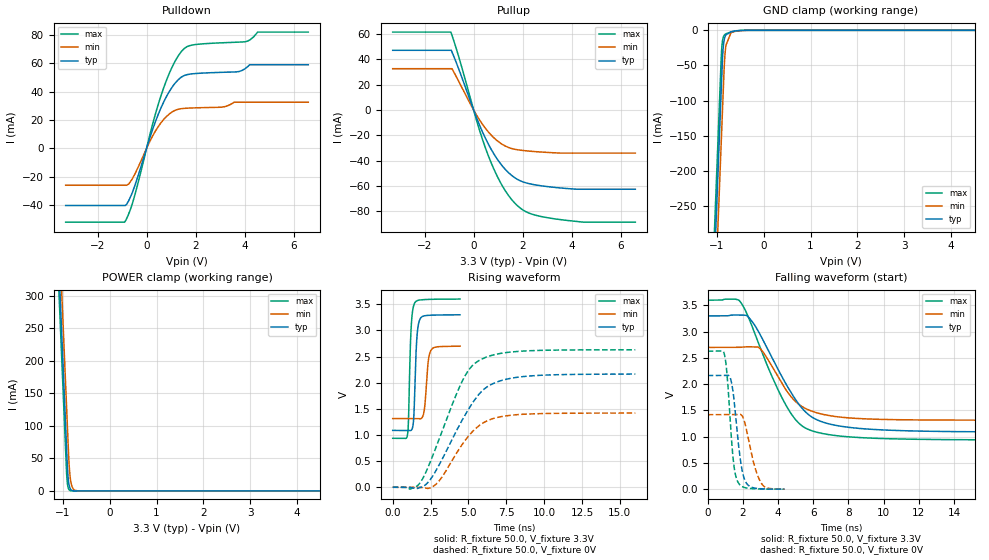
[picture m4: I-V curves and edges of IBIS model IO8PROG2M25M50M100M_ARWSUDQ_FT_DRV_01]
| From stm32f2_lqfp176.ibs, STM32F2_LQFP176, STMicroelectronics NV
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| *** New cell (Generated with 5.14beta1 (Sep 20 2010 13:23:23))
[Model]   IO8PROG2M25M50M100M_ARWSUDQ_FT_DRV_01
Model_type 3-state
Polarity   Non-Inverting
Enable   Active-Low
| CAP_THRESHOLD on pad IOV33 is "CMOS" :
| Rising=10.0% of vddio   Falling=90.0% of vddio
| C_comp min and max val. don't necessarily correlate with the min and max pvt
| but are the smallest and greatest pad capacitance found.
| var   typ   min   max
C_comp   2.32810pF  2.21815pF  2.46460pF
Vmeas = 1.65V   | Reference voltage for timing measurements
Cref  = 50.0pF   | Timing specification test load capacitance value
Rref  = 10.0MOhm   | Timing specification test load resistance value
Vref  = 1.65V   | Timing specification test load voltage
[Model Spec]
| variable   typ   min   max
[Temperature Range] 25.0 125.0 -40.0
| variable   typ   min   max
[Voltage Range] 3.3V 2.7V 3.6V
| variable   typ   min   max
[POWER Clamp Reference] 3.3V 2.7V 3.6V
| variable   typ   min   max
[GND Clamp Reference] 0V 0V 0V
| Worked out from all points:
|   slope of the pulldown table from 0 to 0.495 V, typ, clamps not added: 20 ohm
|   slope of the pullup table from 0 to 0.495 V, typ, clamps not added: 21.7 ohm
|   GND clamp passes 1 mA (typ) near -0.61 V on its own axis
|   POWER clamp passes 1 mA (typ) near -0.81 V on its own axis
|   rising waveform, R_fixture 50.0, V_fixture 3.3V: 20-80 % time 174ps typ, 219ps min, 160ps max; typ from 1.09 V to 3.3 V
|   falling waveform, R_fixture 50.0, V_fixture 3.3V: 20-80 % time 2.28ns typ, 1.77ns min, 2.12ns max; typ from 3.3 V to 1.09 V
|   rising waveform, R_fixture 50.0, V_fixture 0V: 20-80 % time 2.49ns typ, 2.07ns min, 2.18ns max; typ from 0 V to 2.17 V
|   falling waveform, R_fixture 50.0, V_fixture 0V: 20-80 % time 429ps typ, 610ps min, 343ps max; typ from 2.17 V to 0.001 V
[POWER Clamp]
-3.3V     4.11A      4.173A     4.072A
-1.09V    352.5mA    415.9mA    314.5mA
-1.05V    284.5mA    347.9mA    246.5mA
-1.01V    216.5mA    279.9mA    178.5mA
-920mV    63.51mA    126.9mA    25.85mA
-900mV    31.51mA    92.9mA     9.552mA
-890mV    21.35mA    75.9mA     5.807mA
-870mV    9.804mA    44.01mA    2.146mA
-840mV    3.05mA     18.36mA    482.1uA
-780mV    295.2uA    3.194mA    24.34uA
-660mV    2.764uA    96.52uA    62.42nA
6.6V      0A         0A         0A
[GND Clamp]
-3.3V     -4.149A    -4.224A    -4.103A
-1.06V    -341mA     -415.8mA   -295.1mA
-940mV    -137mA     -211.8mA   -91.11mA
-910mV    -86.01mA   -160.8mA   -40.11mA
-900mV    -69.01mA   -143.8mA   -27.13mA
-880mV    -37.2mA    -109.8mA   -14.07mA
-860mV    -20.02mA   -75.82mA   -8.837mA
-840mV    -11.77mA   -45.3mA    -6.542mA
-810mV    -6.468mA   -21.54mA   -4.94mA
-700mV    -2.247mA   -3.206mA   -2.168mA
-470mV    -130uA     -313.8uA   -60.76uA
6.6V      10.47nA    1.304uA    84.25pA
| variable   typ   min   max
[Pullup Reference] 3.3V 2.7V 3.6V
| variable   typ   min   max
[Pulldown Reference] 0V 0V 0V
[Pullup]
-3.3V     46.97mA    32.48mA    61.32mA
-930mV    46.97mA    32.48mA    61.32mA
-880mV    45.6mA     32.48mA    58.74mA
-590mV    31.42mA    21.88mA    40.86mA
240mV     -11.89mA   -7.822mA   -15.87mA
590mV     -26.5mA    -17.07mA   -35.52mA
1.18V     -44.36mA   -27.27mA   -60.11mA
1.54V     -51.43mA   -30.39mA   -70.35mA
1.89V     -55.75mA   -31.69mA   -77.18mA
2.48V     -58.98mA   -32.83mA   -82.75mA
3.6V      -61.62mA   -34.07mA   -86.61mA
6.6V      -62.54mA   -34.07mA   -88.51mA
[Pulldown]
-3.3V     -40.26mA   -25.94mA   -51.99mA
-870mV    -40.25mA   -25.94mA   -51.33mA
-720mV    -36.35mA   -24.93mA   -45.5mA
-470mV    -25.89mA   -17.87mA   -32.39mA
240mV     12.97mA    8.52mA     16.62mA
590mV     28.62mA    18.11mA    37.2mA
1.07V     43.85mA    26mA       58.31mA
1.54V     51.42mA    28.24mA    70.48mA
2.01V     52.82mA    28.63mA    73.27mA
4.01V     56.05mA    32.64mA    75.18mA
4.53V     59mA       32.64mA    82.02mA
6.6V      59mA       32.64mA    82.02mA
[Ramp]
dV/dt_r 1.29886V/2.48885ns 851.30659mV/2.0742ns 1.57728V/2.18503ns
dV/dt_f 1.32782V/2.27584ns 831.60247mV/1.77444ns 1.59819V/2.11818ns
R_load = 50.0
| Removed startup time: 0s 0s 0s  .
| Removed end time: 4.441ns.
[Rising Waveform]
R_fixture   = 50.0
V_fixture   = 3.3V
V_fixture_min = 2.7V
V_fixture_max = 3.6V
0s        1.087V     1.314V     936.3mV
980ps     1.087V     1.314V     1.006V
1.042ns   1.086V     1.314V     1.284V
1.208ns   1.086V     1.314V     3V
1.429ns   1.589V     1.314V     3.511V
1.587ns   2.822V     1.313V     3.564V
1.809ns   3.219V     1.309V     3.581V
2.085ns   3.278V     1.472V     3.588V
2.521ns   3.29V      2.617V     3.594V
4.443ns   3.298V     2.698V     3.598V
| Removed startup time: 0s 0s 0s  .
| Removed end time: 20.415ns.
[Falling Waveform]
R_fixture   = 50.0
V_fixture   = 3.3V
V_fixture_min = 2.7V
V_fixture_max = 3.6V
0s        3.3V       2.7V       3.6V
1.83ns    3.315V     2.701V     3.579V
2.28ns    3.29V      2.711V     3.304V
2.955ns   2.962V     2.685V     2.725V
4.335ns   2.073V     1.953V     1.67V
5.02ns    1.694V     1.661V     1.315V
5.735ns   1.419V     1.51V      1.135V
6.95ns    1.239V     1.399V     1.036V
9.1ns     1.144V     1.337V     975.1mV
20.43ns   1.087V     1.314V     936.6mV
| Removed startup time: 0s 0s 0s  .
| Removed end time: 16.01ns.
[Rising Waveform]
R_fixture   = 50.0
V_fixture   = 0V
V_fixture_min = 0V
V_fixture_max = 0V
0s        8.041nV    322.2nV    5.734nV
1.14ns    -513.1uV   -6.917uV   -36.27mV
1.85ns    -3.412mV   -2.228mV   102.7mV
2.345ns   97.24mV    -22.08mV   389.7mV
2.97ns    376.1mV    89.52mV    846.8mV
4.63ns    1.306V     835.3mV    2.051V
5.79ns    1.809V     1.195V     2.439V
6.75ns    1.999V     1.324V     2.538V
8.385ns   2.109V     1.391V     2.6V
16.02ns   2.165V     1.419V     2.629V
| Removed startup time: 0s 0s 0s  .
| Removed end time: 4.359ns.
[Falling Waveform]
R_fixture   = 50.0
V_fixture   = 0V
V_fixture_min = 0V
V_fixture_max = 0V
0s        2.165V     1.419V     2.629V
965ps     2.166V     1.419V     2.552V
1.146ns   2.171V     1.419V     2.02V
1.364ns   2.019V     1.418V     910.9mV
1.525ns   1.619V     1.42V      375.3mV
1.734ns   906.5mV    1.425V     127.9mV
1.976ns   332.1mV    1.389V     47.53mV
2.277ns   84.61mV    1.02V      19.85mV
3.04ns    7.655mV    119mV      3.112mV
4.361ns   1.031mV    1.529mV    697.7uV
